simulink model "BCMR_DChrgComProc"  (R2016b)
settings: Solver=FixedStepDiscrete  StartTime=0.0  StopTime=10.0  FixedStep=0.01  RelTol=1e-3  EnableMultiTasking=on
undefined symbols (not defined in the file or in its folder): BCMR_ahBattRatdCpctyBrm_C, BCMR_BattSocErrBsmEna_C, BCMR_eBattRatedEnrgBcp_C, BCMR_G1E0PlatformSwCom_C, BCMR_iMaxChrgCurrPmtdBcp_C, BCMR_numBattTypeBrm_C, BCMR_numComVer2011Brm_C, BCMR_numComVer2015Brm_C, BCMR_tMaxTempPmtdBcp_C, BCMR_uBattRatdPackVoltBcp_C, BCMR_uBattRatdPackVoltBrm_C, BCMR_uMaxChrgCellVoltPmtdBcp_C, BCMR_uMaxPmtDChrgVolt_C
libraries: simulink x32
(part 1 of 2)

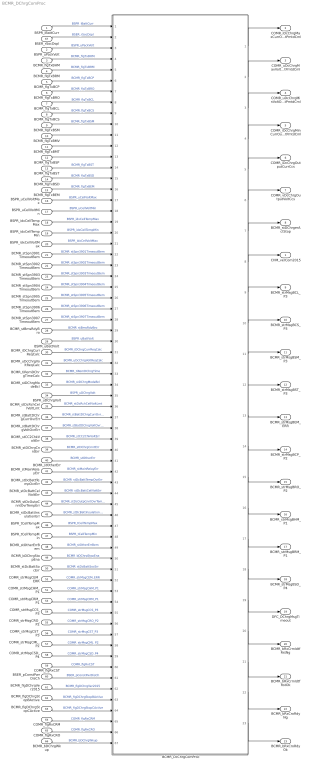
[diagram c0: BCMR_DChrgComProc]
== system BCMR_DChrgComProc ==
  BSPR_iBattCurr : Inport
  BSPR_uPackVolt : Inport  Port=2
  BCMR_flgTxBHM : Inport  Port=3
  BCMR_flgTxBRM : Inport  Port=4
  BCMR_flgTxBCP : Inport  Port=5
  BCMR_flgTxBRO : Inport  Port=6
  BCMR_flgTxBCL : Inport  Port=7
  BCMR_flgTxBCS : Inport  Port=8
  BCMR_flgTxBSM : Inport  Port=9
  BCMR_flgTxBMV : Inport  Port=10
  BCMR_flgTxBMT : Inport  Port=11
  BCMR_flgTxBSP : Inport  Port=12
  BCMR_flgTxBST : Inport  Port=13
  BCMR_flgTxBSD : Inport  Port=14
  BCMR_flgTxBEM : Inport  Port=15
  BSPR_uCellVoltMax : Inport  Port=16
  BSPR_uCellVoltMin : Inport  Port=17
  BSPR_idxCellTempMax : Inport  Port=18
  BSPR_idxCellTempMin : Inport  Port=19
  BSPR_idxCellVoltMax : Inport  Port=20
  BCMR_stSpn3901TimeoutBem : Inport  Port=21
  BCMR_stSpn3902TimeoutBem : Inport  Port=22
  BCMR_stSpn3903TimeoutBem : Inport  Port=23
  BCMR_stSpn3904TimeoutBem : Inport  Port=24
  BCMR_stSpn3905TimeoutBem : Inport  Port=25
  BCMR_stSpn3906TimeoutBem : Inport  Port=26
  BCMR_stSpn3907TimeoutBem : Inport  Port=27
  BCMR_stBmsRdyBro : Inport  Port=28
  BSPR_uBattVolt : Inport  Port=29
  BCMR_iDChrgCurrReqCalc : Inport  Port=30
  BCMR_uDcChrgVoltReqCalc : Inport  Port=31
  BCMR_tiRemDChrgTimeCalc : Inport  Port=32
  BCMR_stDChrgModeBcl : Inport  Port=33
  BSPR_uDChrgVolt : Inport  Port=34
  BCMR_stDcRchCellVoltLmt : Inport  Port=35
  BCMR_stBattDChrgCurrOvrErr : Inport  Port=36
  BCMR_stBattDChrgVoltOvrErr : Inport  Port=37
  BCMR_stCC2ChkVoltErr : Inport  Port=38
  BCMR_stDChrgCnntErr : Inport  Port=39
  BCMR_stOtherErr : Inport  Port=40
  BCMR_stMainRelayErr : Inport  Port=41
  BCMR_stDcBattTempOvrErr : Inport  Port=42
  BCMR_stDcBattCellVoltErr : Inport  Port=43
  BCMR_stDcOutpCnntOvrTempErr : Inport  Port=44
  BCMR_stDcBattInsulationErr : Inport  Port=45
  BSPR_tCellTempMax : Inport  Port=46
  BSPR_tCellTempMin : Inport  Port=47
  BCMR_stOtherErrBem : Inport  Port=48
  BCMR_bDChrgStopEna : Inport  Port=49
  BCMR_stDcBattSocErr : Inport  Port=50
  COMR_strMsgCHM_P1 : Inport  Port=51  OutDataTypeStr=Bus: MSG_CHM_P1
  COMR_strMsgCEM_ERR : Inport  Port=52  OutDataTypeStr=Bus: MSG_CEM_ERR
  COMR_strMsgCRM_P1 : Inport  Port=53  OutDataTypeStr=Bus: MSG_CRM_P1
  COMR_strMsgCCS_P3 : Inport  Port=54  OutDataTypeStr=Bus: MSG_CCS_P3
  COMR_strMsgCRO_P2 : Inport  Port=55  OutDataTypeStr=Bus: MSG_CRO_P2
  COMR_strMsgCST_P3 : Inport  Port=56  OutDataTypeStr=Bus: MSG_CST_P3
  COMR_strMsgCML_P2 : Inport  Port=57  OutDataTypeStr=Bus: MSG_CML_P2
  COMR_strMsgCSD_P4 : Inport  Port=58  OutDataTypeStr=Bus: MSG_CSD_P4
  COMR_flgRxCST : Inport  Port=59
  BSER_pConstPwrDisCh : Inport  Port=60
  BCMR_flgDChrgVer2015 : Inport  Port=61
  BCMR_flgDChrgStopBActive : Inport  Port=62
  BCMR_flgDChrgStopCActive : Inport  Port=63
  COMR_flgRxCRM : Inport  Port=64
  COMR_flgRxCRO : Inport  Port=65
  BCMR_bDChrgWkup : Inport  Port=66
  BSER_rSocDspl : Inport  Port=67
  BCMR_DcChrgComProc : Subsystem
  CHM_verCom2015 : Outport
  COMR_iDcChrgMaxCurrOutputPmtdCml : Outport  Port=2
  COMR_uDcChrgMaxVoltOutputPmtdCml : Outport  Port=3
  COMR_uDcChrgMinVoltOutputPmtdCml : Outport  Port=4
  COMR_iDcChrgMinCurrOutputPmtdCml : Outport  Port=5
  COMR_iDcChrgOutputCurrCcs : Outport  Port=6
  COMR_vDcChrgOutputVoltCcs : Outport  Port=7
  BCMR_stDChrgerActStop : Outport  Port=8
  BCMR_strMsgBCL_P3 : Outport  Port=9  OutDataTypeStr=Bus: MSG_BCL_P3
  BCMR_strMsgBCS_P3 : Outport  Port=10  OutDataTypeStr=Bus: MSG_BCS_P3
  BCMR_strMsgBSM_P3 : Outport  Port=11  OutDataTypeStr=Bus: MSG_BSM_P3
  BCMR_strMsgBST_P3 : Outport  Port=12  OutDataTypeStr=Bus: MSG_BST_P3
  BCMR_strMsgBEM_ERR : Outport  Port=13  OutDataTypeStr=Bus: MSG_BEM_ERR
  BCMR_strMsgBCP_P2 : Outport  Port=14  OutDataTypeStr=Bus: MSG_BCP_P2
  BCMR_strMsgBRO_P2 : Outport  Port=15  OutDataTypeStr=Bus: MSG_BRO_P2
  BCMR_strMsgBHM_P1 : Outport  Port=16  OutDataTypeStr=Bus: MSG_BHM_P1
  BCMR_strMsgBRM_P1 : Outport  Port=17  OutDataTypeStr=Bus: MSG_BRM_P1
  BCMR_strMsgBSD_P4 : Outport  Port=18  OutDataTypeStr=Bus: MSG_BSD_P4
  DFC_DChrgMsgTimeout : Outport  Port=19
  BCMR_bRxCrmIdtfRstNg : Outport  Port=20
  BCMR_bRxCrmIdtfRstOk : Outport  Port=21
  BCMR_bRxCroRdyNg : Outport  Port=22
  BCMR_bRxCroRdyOk : Outport  Port=23
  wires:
  BSPR_iBattCurr/1 -> BCMR_DcChrgComProc/1(BSPR_iBattCurr)  "BSPR_iBattCurr"
  BSPR_uPackVolt/1 -> BCMR_DcChrgComProc/3(BSPR_uPackVolt)  "BSPR_uPackVolt"
  BCMR_flgTxBHM/1 -> BCMR_DcChrgComProc/4(BCMR_flgTxBHM)  "BCMR_flgTxBHM"
  BCMR_flgTxBRM/1 -> BCMR_DcChrgComProc/5(BCMR_flgTxBRM)  "BCMR_flgTxBRM"
  BCMR_flgTxBCP/1 -> BCMR_DcChrgComProc/6(BCMR_flgTxBCP)  "BCMR_flgTxBCP"
  BCMR_flgTxBRO/1 -> BCMR_DcChrgComProc/7(BCMR_flgTxBRO)  "BCMR_flgTxBRO"
  BCMR_flgTxBCL/1 -> BCMR_DcChrgComProc/8(BCMR_flgTxBCL)  "BCMR_flgTxBCL"
  BCMR_flgTxBCS/1 -> BCMR_DcChrgComProc/9(BCMR_flgTxBCS)  "BCMR_flgTxBCS"
  BCMR_flgTxBSM/1 -> BCMR_DcChrgComProc/10(BCMR_flgTxBSM)  "BCMR_flgTxBSM"
  BCMR_flgTxBMV/1 -> BCMR_DcChrgComProc/11(BCMR_flgTxBMV)
  BCMR_flgTxBMT/1 -> BCMR_DcChrgComProc/12(BCMR_flgTxBMT)
  BCMR_flgTxBSP/1 -> BCMR_DcChrgComProc/13(BCMR_flgTxBSP)
  BCMR_flgTxBST/1 -> BCMR_DcChrgComProc/14(BCMR_flgTxBST)  "BCMR_flgTxBST"
  BCMR_flgTxBSD/1 -> BCMR_DcChrgComProc/15(BCMR_flgTxBSD)  "BCMR_flgTxBSD"
  BCMR_flgTxBEM/1 -> BCMR_DcChrgComProc/16(BCMR_flgTxBEM)  "BCMR_flgTxBEM"
  BSPR_uCellVoltMax/1 -> BCMR_DcChrgComProc/17(BSPR_uCellVoltMax)  "BSPR_uCellVoltMax"
  BSPR_uCellVoltMin/1 -> BCMR_DcChrgComProc/18(BSPR_uCellVoltMin)  "BSPR_uCellVoltMin"
  BSPR_idxCellTempMax/1 -> BCMR_DcChrgComProc/19(BSPR_idxBattTempMax)  "BSPR_idxCellTempMax"
  BSPR_idxCellTempMin/1 -> BCMR_DcChrgComProc/20(BSPR_idxBattTempMin)  "BSPR_idxCellTempMin"
  BSPR_idxCellVoltMax/1 -> BCMR_DcChrgComProc/21(BSPR_idxCellVoltMax)  "BSPR_idxCellVoltMax"
  BCMR_stSpn3901TimeoutBem/1 -> BCMR_DcChrgComProc/22(BCMR_stSpn3901TimeoutBem)  "BCMR_stSpn3901TimeoutBem"
  BCMR_stSpn3902TimeoutBem/1 -> BCMR_DcChrgComProc/23(BCMR_stSpn3902TimeoutBem)  "BCMR_stSpn3902TimeoutBem"
  BCMR_stSpn3903TimeoutBem/1 -> BCMR_DcChrgComProc/24(BCMR_stSpn3903TimeoutBem)  "BCMR_stSpn3903TimeoutBem"
  BCMR_stSpn3904TimeoutBem/1 -> BCMR_DcChrgComProc/25(BCMR_stSpn3904TimeoutBem)  "BCMR_stSpn3904TimeoutBem"
  BCMR_stSpn3905TimeoutBem/1 -> BCMR_DcChrgComProc/26(BCMR_stSpn3905TimeoutBem)  "BCMR_stSpn3905TimeoutBem"
  BCMR_stSpn3906TimeoutBem/1 -> BCMR_DcChrgComProc/27(BCMR_stSpn3906TimeoutBem)  "BCMR_stSpn3906TimeoutBem"
  BCMR_stSpn3907TimeoutBem/1 -> BCMR_DcChrgComProc/28(BCMR_stSpn3907TimeoutBem)  "BCMR_stSpn3907TimeoutBem"
  BCMR_stBmsRdyBro/1 -> BCMR_DcChrgComProc/29(BCMR_stBmsRdyBro)  "BCMR_stBmsRdyBro"
  BSPR_uBattVolt/1 -> BCMR_DcChrgComProc/30(BSPR_uBattVolt)  "BSPR_uBattVolt"
  BCMR_iDChrgCurrReqCalc/1 -> BCMR_DcChrgComProc/31(BCMR_iDChrgCurrReqCalc)  "BCMR_iDChrgCurrReqCalc"
  BCMR_uDcChrgVoltReqCalc/1 -> BCMR_DcChrgComProc/32(BCMR_uDcChrgVoltReqCalc)  "BCMR_uDcChrgVoltReqCalc"
  BCMR_tiRemDChrgTimeCalc/1 -> BCMR_DcChrgComProc/33(BCMR_tiRemDChrgTime)  "BCMR_tiRemDChrgTime"
  BCMR_stDChrgModeBcl/1 -> BCMR_DcChrgComProc/34(BCMR_stDChrgModeBcl)  "BCMR_stDChrgModeBcl"
  BSPR_uDChrgVolt/1 -> BCMR_DcChrgComProc/35(BSPR_uDChrgVolt)  "BSPR_uDChrgVolt"
  BCMR_stDcRchCellVoltLmt/1 -> BCMR_DcChrgComProc/36(BCMR_stDcRchCellVoltLmt)  "BCMR_stDcRchCellVoltLmt"
  BCMR_stBattDChrgCurrOvrErr/1 -> BCMR_DcChrgComProc/37(BCMR_stBattDChrgCurrOvrErr)  "BCMR_stBattDChrgCurrOvrErr"
  BCMR_stBattDChrgVoltOvrErr/1 -> BCMR_DcChrgComProc/38(BCMR_stBattDChrgVoltOvrErr)  "BCMR_stBattDChrgVoltOvrErr"
  BCMR_stCC2ChkVoltErr/1 -> BCMR_DcChrgComProc/39(BCMR_stCC2ChkVoltErr)  "BCMR_stCC2ChkVoltErr"
  BCMR_stDChrgCnntErr/1 -> BCMR_DcChrgComProc/40(BCMR_stDChrgCnntErr)  "BCMR_stDChrgCnntErr"
  BCMR_stOtherErr/1 -> BCMR_DcChrgComProc/41(BCMR_stOtherErr)  "BCMR_stOtherErr"
  BCMR_stMainRelayErr/1 -> BCMR_DcChrgComProc/42(BCMR_stMainRelayErr)  "BCMR_stMainRelayErr"
  BCMR_stDcBattTempOvrErr/1 -> BCMR_DcChrgComProc/43(BCMR_stDcBattTempOvrErr)  "BCMR_stDcBattTempOvrErr"
  BCMR_stDcBattCellVoltErr/1 -> BCMR_DcChrgComProc/44(BCMR_stDcBattCellVoltErr)  "BCMR_stDcBattCellVoltErr"
  BCMR_stDcOutpCnntOvrTempErr/1 -> BCMR_DcChrgComProc/45(BCMR_stDcOutpCnntOvrTempErr)  "BCMR_stDcOutpCnntOvrTempErr"
  BCMR_stDcBattInsulationErr/1 -> BCMR_DcChrgComProc/46(BCMR_stDcBattInsulationErr)  "BCMR_stDcBattInsulationErr"
  BSPR_tCellTempMax/1 -> BCMR_DcChrgComProc/47(BSPR_tBattTempMax)  "BSPR_tCellTempMax"
  BSPR_tCellTempMin/1 -> BCMR_DcChrgComProc/48(BSPR_tBattTempMin)  "BSPR_tCellTempMin"
  BCMR_DcChrgComProc/1(COMR_iDcChrgMaxCurrOutputPmtdCml) -> COMR_iDcChrgMaxCurrOutputPmtdCml/1
  BCMR_DcChrgComProc/2(COMR_uDcChrgMaxVoltOutputPmtdCml) -> COMR_uDcChrgMaxVoltOutputPmtdCml/1
  BCMR_DcChrgComProc/3(COMR_uDcChrgMinVoltOutputPmtdCml) -> COMR_uDcChrgMinVoltOutputPmtdCml/1
  BCMR_DcChrgComProc/4(COMR_iDcChrgMinCurrOutputPmtdCml) -> COMR_iDcChrgMinCurrOutputPmtdCml/1
  BCMR_DcChrgComProc/5(COMR_iDcChrgOutputCurrCcs) -> COMR_iDcChrgOutputCurrCcs/1
  BCMR_DcChrgComProc/6(COMR_vDcChrgOutputVoltCcs) -> COMR_vDcChrgOutputVoltCcs/1
  BCMR_DcChrgComProc/7(BCMR_stDChrgerActStop) -> BCMR_stDChrgerActStop/1
  BCMR_stOtherErrBem/1 -> BCMR_DcChrgComProc/49(BCMR_stOtherErrBem)  "BCMR_stOtherErrBem"
  BCMR_DcChrgComProc/8(BCMR_verDChrgCom2015) -> CHM_verCom2015/1
  BCMR_bDChrgStopEna/1 -> BCMR_DcChrgComProc/50(BCMR_bDChrgStopEna)  "BCMR_bDChrgStopEna"
  BCMR_stDcBattSocErr/1 -> BCMR_DcChrgComProc/51(BCMR_stDcBattSocErr)  "BCMR_stDcBattSocErr"
  COMR_strMsgCSD_P4/1 -> BCMR_DcChrgComProc/59(COMR_strRxCSD)  "COMR_strMsgCSD_P4"
  COMR_strMsgCML_P2/1 -> BCMR_DcChrgComProc/58(COMR_strRxCML)  "COMR_strMsgCML_P2"
  COMR_strMsgCST_P3/1 -> BCMR_DcChrgComProc/57(COMR_strRxCST)  "COMR_strMsgCST_P3"
  COMR_strMsgCRO_P2/1 -> BCMR_DcChrgComProc/56(COMR_strRxCRO)  "COMR_strMsgCRO_P2"
  COMR_strMsgCCS_P3/1 -> BCMR_DcChrgComProc/55(COMR_strRxCCS)  "COMR_strMsgCCS_P3"
  COMR_strMsgCRM_P1/1 -> BCMR_DcChrgComProc/54(COMR_strRxCRM)  "COMR_strMsgCRM_P1"
  COMR_strMsgCEM_ERR/1 -> BCMR_DcChrgComProc/52(COMR_strRxCEM)  "COMR_strMsgCEM_ERR"
  COMR_strMsgCHM_P1/1 -> BCMR_DcChrgComProc/53(COMR_strRxCHM)  "COMR_strMsgCHM_P1"
  BCMR_DcChrgComProc/9(BCMR_strMsgBCL_P3) -> BCMR_strMsgBCL_P3/1
  BCMR_DcChrgComProc/10(BCMR_strMsgBCS_P3) -> BCMR_strMsgBCS_P3/1
  BCMR_DcChrgComProc/11(BCMR_strMsgBSM_P3) -> BCMR_strMsgBSM_P3/1
  BCMR_DcChrgComProc/12(BCMR_strMsgBST_P3) -> BCMR_strMsgBST_P3/1
  BCMR_DcChrgComProc/13(BCMR_strMsgBEM_ERR) -> BCMR_strMsgBEM_ERR/1
  BCMR_DcChrgComProc/14(BCMR_strMsgBCP_P2) -> BCMR_strMsgBCP_P2/1
  BCMR_DcChrgComProc/15(BCMR_strMsgBRO_P2) -> BCMR_strMsgBRO_P2/1
  BCMR_DcChrgComProc/16(BCMR_strMsgBHM_P1) -> BCMR_strMsgBHM_P1/1
  BCMR_DcChrgComProc/17(BCMR_strMsgBRM_P1) -> BCMR_strMsgBRM_P1/1
  BCMR_DcChrgComProc/18(BCMR_strMsgBSD_P4) -> BCMR_strMsgBSD_P4/1
  BCMR_DcChrgComProc/19(DFC_DChrgMsgTimeout) -> DFC_DChrgMsgTimeout/1
  COMR_flgRxCST/1 -> BCMR_DcChrgComProc/60(COMR_flgRxCST)  "COMR_flgRxCST"
  BSER_pConstPwrDisCh/1 -> BCMR_DcChrgComProc/61(BSER_pConstPwrDisCh)  "BSER_pConstPwrDisCh"
  BCMR_flgDChrgVer2015/1 -> BCMR_DcChrgComProc/62(BCMR_flgDChrgVer2015)  "BCMR_flgDChrgVer2015"
  BCMR_flgDChrgStopBActive/1 -> BCMR_DcChrgComProc/63(BCMR_flgDChrgStopBActive)  "BCMR_flgDChrgStopBActive"
  BCMR_flgDChrgStopCActive/1 -> BCMR_DcChrgComProc/64(BCMR_flgDChrgStopCActive)  "BCMR_flgDChrgStopCActive"
  COMR_flgRxCRM/1 -> BCMR_DcChrgComProc/65(COMR_flgRxCRM)  "COMR_flgRxCRM"
  COMR_flgRxCRO/1 -> BCMR_DcChrgComProc/66(COMR_flgRxCRO)  "COMR_flgRxCRO"
  BCMR_DcChrgComProc/20(BCMR_bRxCrmIdtfRstNg) -> BCMR_bRxCrmIdtfRstNg/1
  BCMR_DcChrgComProc/21(BCMR_bRxCrmIdtfRstOk) -> BCMR_bRxCrmIdtfRstOk/1
  BCMR_DcChrgComProc/23(BCMR_bRxCroRdyOk) -> BCMR_bRxCroRdyOk/1
  BCMR_DcChrgComProc/22(BCMR_bRxCroRdyNg) -> BCMR_bRxCroRdyNg/1
  BCMR_bDChrgWkup/1 -> BCMR_DcChrgComProc/67(BCMR_bDChrgWkup)  "BCMR_bDChrgWkup"
  BSER_rSocDspl/1 -> BCMR_DcChrgComProc/2(BSER_rSocDspl)  "BSER_rSocDspl"

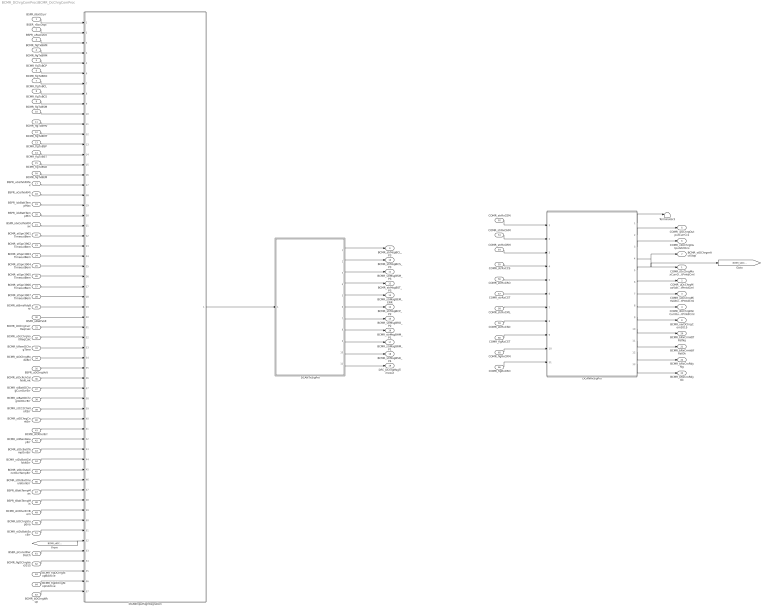
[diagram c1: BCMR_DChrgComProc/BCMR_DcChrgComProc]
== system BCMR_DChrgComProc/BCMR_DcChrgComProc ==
  BSPR_iBattCurr : Inport
  BSER_rSocDspl : Inport  Port=2
  BSPR_uPackVolt : Inport  Port=3
  BCMR_flgTxBHM : Inport  Port=4
  BCMR_flgTxBRM : Inport  Port=5
  BCMR_flgTxBCP : Inport  Port=6
  BCMR_flgTxBRO : Inport  Port=7
  BCMR_flgTxBCL : Inport  Port=8
  BCMR_flgTxBCS : Inport  Port=9
  BCMR_flgTxBSM : Inport  Port=10
  BCMR_flgTxBMV : Inport  Port=11
  BCMR_flgTxBMT : Inport  Port=12
  BCMR_flgTxBSP : Inport  Port=13
  BCMR_flgTxBST : Inport  Port=14
  BCMR_flgTxBSD : Inport  Port=15
  BCMR_flgTxBEM : Inport  Port=16
  BSPR_uCellVoltMax : Inport  Port=17
  BSPR_uCellVoltMin : Inport  Port=18
  BSPR_idxBattTempMax : Inport  Port=19
  BSPR_idxBattTempMin : Inport  Port=20
  BSPR_idxCellVoltMax : Inport  Port=21
  BCMR_stSpn3901TimeoutBem : Inport  Port=22
  BCMR_stSpn3902TimeoutBem : Inport  Port=23
  BCMR_stSpn3903TimeoutBem : Inport  Port=24
  BCMR_stSpn3904TimeoutBem : Inport  Port=25
  BCMR_stSpn3905TimeoutBem : Inport  Port=26
  BCMR_stSpn3906TimeoutBem : Inport  Port=27
  BCMR_stSpn3907TimeoutBem : Inport  Port=28
  BCMR_stBmsRdyBro : Inport  Port=29
  BSPR_uBattVolt : Inport  Port=30
  BCMR_iDChrgCurrReqCalc : Inport  Port=31
  BCMR_uDcChrgVoltReqCalc : Inport  Port=32
  BCMR_tiRemDChrgTime : Inport  Port=33
  BCMR_stDChrgModeBcl : Inport  Port=34
  BSPR_uDChrgVolt : Inport  Port=35
  BCMR_stDcRchCellVoltLmt : Inport  Port=36
  BCMR_stBattDChrgCurrOvrErr : Inport  Port=37
  BCMR_stBattDChrgVoltOvrErr : Inport  Port=38
  BCMR_stCC2ChkVoltErr : Inport  Port=39
  BCMR_stDChrgCnntErr : Inport  Port=40
  BCMR_stOtherErr : Inport  Port=41
  BCMR_stMainRelayErr : Inport  Port=42
  BCMR_stDcBattTempOvrErr : Inport  Port=43
  BCMR_stDcBattCellVoltErr : Inport  Port=44
  BCMR_stDcOutpCnntOvrTempErr : Inport  Port=45
  BCMR_stDcBattInsulationErr : Inport  Port=46
  BSPR_tBattTempMax : Inport  Port=47
  BSPR_tBattTempMin : Inport  Port=48
  BCMR_stOtherErrBem : Inport  Port=49
  BCMR_bDChrgStopEna : Inport  Port=50
  BCMR_stDcBattSocErr : Inport  Port=51
  COMR_strRxCEM : Inport  Port=52  OutDataTypeStr=Bus: MSG_CEM_ERR
  COMR_strRxCHM : Inport  Port=53  OutDataTypeStr=Bus: MSG_CHM_P1
  COMR_strRxCRM : Inport  Port=54  OutDataTypeStr=Bus: MSG_CRM_P1
  COMR_strRxCCS : Inport  Port=55  OutDataTypeStr=Bus: MSG_CCS_P3
  COMR_strRxCRO : Inport  Port=56  OutDataTypeStr=Bus: MSG_CRO_P2
  COMR_strRxCST : Inport  Port=57  OutDataTypeStr=Bus: MSG_CST_P3
  COMR_strRxCML : Inport  Port=58  OutDataTypeStr=Bus: MSG_CML_P2
  COMR_strRxCSD : Inport  Port=59  OutDataTypeStr=Bus: MSG_CSD_P4
  COMR_flgRxCST : Inport  Port=60
  BSER_pConstPwrDisCh : Inport  Port=61
  BCMR_flgDChrgVer2015 : Inport  Port=62
  BCMR_flgDChrgStopBActive : Inport  Port=63
  BCMR_flgDChrgStopCActive : Inport  Port=64
  COMR_flgRxCRM : Inport  Port=65
  COMR_flgRxCRO : Inport  Port=66
  BCMR_bDChrgWkup : Inport  Port=67
  DCANInputSigIntegration : Subsystem
  DCANRxSigPro : Subsystem
  DCANTxSigPro : Subsystem
  Terminator3 : Terminator
  COMR_iDcChrgMaxCurrOutputPmtdCml : Outport
  COMR_uDcChrgMaxVoltOutputPmtdCml : Outport  Port=2
  COMR_uDcChrgMinVoltOutputPmtdCml : Outport  Port=3
  COMR_iDcChrgMinCurrOutputPmtdCml : Outport  Port=4
  COMR_iDcChrgOutputCurrCcs : Outport  Port=5
  COMR_vDcChrgOutputVoltCcs : Outport  Port=6
  BCMR_stDChrgerActStop : Outport  Port=7
  BCMR_verDChrgCom2015 : Outport  Port=8
  BCMR_strMsgBCL_P3 : Outport  Port=9  OutDataTypeStr=Bus: MSG_BCL_P3
  BCMR_strMsgBCS_P3 : Outport  Port=10  OutDataTypeStr=Bus: MSG_BCS_P3
  BCMR_strMsgBSM_P3 : Outport  Port=11  OutDataTypeStr=Bus: MSG_BSM_P3
  BCMR_strMsgBST_P3 : Outport  Port=12  OutDataTypeStr=Bus: MSG_BST_P3
  BCMR_strMsgBEM_ERR : Outport  Port=13  OutDataTypeStr=Bus: MSG_BEM_ERR
  BCMR_strMsgBCP_P2 : Outport  Port=14  OutDataTypeStr=Bus: MSG_BCP_P2
  BCMR_strMsgBRO_P2 : Outport  Port=15  OutDataTypeStr=Bus: MSG_BRO_P2
  BCMR_strMsgBHM_P1 : Outport  Port=16  OutDataTypeStr=Bus: MSG_BHM_P1
  BCMR_strMsgBRM_P1 : Outport  Port=17  OutDataTypeStr=Bus: MSG_BRM_P1
  BCMR_strMsgBSD_P4 : Outport  Port=18  OutDataTypeStr=Bus: MSG_BSD_P4
  DFC_DChrgMsgTimeout : Outport  Port=19
  BCMR_bRxCrmIdtfRstNg : Outport  Port=20
  BCMR_bRxCrmIdtfRstOk : Outport  Port=21
  BCMR_bRxCroRdyNg : Outport  Port=22
  BCMR_bRxCroRdyOk : Outport  Port=23
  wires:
  COMR_strRxCEM/1 -> DCANRxSigPro/1(COMR_strRxCEM)
  COMR_strRxCHM/1 -> DCANRxSigPro/2(COMR_strRxCHM)
  COMR_strRxCRM/1 -> DCANRxSigPro/3(COMR_strRxCRM)
  COMR_strRxCCS/1 -> DCANRxSigPro/4(COMR_strRxCCS)
  COMR_strRxCRO/1 -> DCANRxSigPro/5(COMR_strRxCRO)
  COMR_strRxCST/1 -> DCANRxSigPro/6(COMR_strRxCST)
  COMR_strRxCML/1 -> DCANRxSigPro/7(COMR_strRxCML)
  COMR_strRxCSD/1 -> DCANRxSigPro/8(COMR_strRxCSD)
  DCANRxSigPro/2(COMR_iDcChrgOutputCurrCcs) -> COMR_iDcChrgOutputCurrCcs/1
  DCANRxSigPro/3(COMR_vDcChrgOutputVoltCcs) -> COMR_vDcChrgOutputVoltCcs/1
  DCANRxSigPro/4(BCMR_stDChrgerActStop) -> [BCMR_stDChrgerActStop], BCMR_stDChrgerActStop/1
  DCANRxSigPro/5(COMR_iDcChrgMaxCurrOutputPmtdCml) -> COMR_iDcChrgMaxCurrOutputPmtdCml/1
  DCANRxSigPro/6(COMR_uDcChrgMaxVoltOutputPmtdCml) -> COMR_uDcChrgMaxVoltOutputPmtdCml/1
  DCANRxSigPro/7(COMR_uDcChrgMinVoltOutputPmtdCml) -> COMR_uDcChrgMinVoltOutputPmtdCml/1
  DCANRxSigPro/8(COMR_iDcChrgMinCurrOutputPmtdCml) -> COMR_iDcChrgMinCurrOutputPmtdCml/1
  DCANRxSigPro/9(BCMR_verDChrgCom2015) -> BCMR_verDChrgCom2015/1
  BSPR_iBattCurr/1 -> DCANInputSigIntegration/1(BSPR_iBattCurr)
  BSER_rSocDspl/1 -> DCANInputSigIntegration/2(BSER_rSocDspl)
  BSPR_uPackVolt/1 -> DCANInputSigIntegration/3(BSPR_uPackVolt)
  BCMR_flgTxBHM/1 -> DCANInputSigIntegration/4(BCMR_flgTxBHM)
  BCMR_flgTxBRM/1 -> DCANInputSigIntegration/5(BCMR_flgTxBRM)
  BCMR_flgTxBCP/1 -> DCANInputSigIntegration/6(BCMR_flgTxBCP)
  BCMR_flgTxBRO/1 -> DCANInputSigIntegration/7(BCMR_flgTxBRO)
  BCMR_flgTxBCL/1 -> DCANInputSigIntegration/8(BCMR_flgTxBCL)
  BCMR_flgTxBCS/1 -> DCANInputSigIntegration/9(BCMR_flgTxBCS)
  BCMR_flgTxBSM/1 -> DCANInputSigIntegration/10(BCMR_flgTxBSM)
  BCMR_flgTxBMV/1 -> DCANInputSigIntegration/11(BCMR_flgTxBMV)
  BCMR_flgTxBMT/1 -> DCANInputSigIntegration/12(BCMR_flgTxBMT)
  BCMR_flgTxBSP/1 -> DCANInputSigIntegration/13(BCMR_flgTxBSP)
  BCMR_flgTxBST/1 -> DCANInputSigIntegration/14(BCMR_flgTxBST)
  BCMR_flgTxBSD/1 -> DCANInputSigIntegration/15(BCMR_flgTxBSD)
  BCMR_flgTxBEM/1 -> DCANInputSigIntegration/16(BCMR_flgTxBEM)
  BSPR_uCellVoltMax/1 -> DCANInputSigIntegration/17(BSPR_uCellVoltMax)
  BSPR_uCellVoltMin/1 -> DCANInputSigIntegration/18(BSPR_uCellVoltMin)
  BSPR_idxBattTempMax/1 -> DCANInputSigIntegration/19(BSPR_idxBattTempMax)
  BSPR_idxBattTempMin/1 -> DCANInputSigIntegration/20(BSPR_idxBattTempMin)
  BSPR_idxCellVoltMax/1 -> DCANInputSigIntegration/21(BSPR_idxCellVoltMax)
  BCMR_stSpn3901TimeoutBem/1 -> DCANInputSigIntegration/22(BCMR_stSpn3901TimeoutBem)
  BCMR_stSpn3902TimeoutBem/1 -> DCANInputSigIntegration/23(BCMR_stSpn3902TimeoutBem)
  BCMR_stSpn3903TimeoutBem/1 -> DCANInputSigIntegration/24(BCMR_stSpn3903TimeoutBem)
  BCMR_stSpn3904TimeoutBem/1 -> DCANInputSigIntegration/25(BCMR_stSpn3904TimeoutBem)
  BCMR_stSpn3905TimeoutBem/1 -> DCANInputSigIntegration/26(BCMR_stSpn3905TimeoutBem)
  BCMR_stSpn3906TimeoutBem/1 -> DCANInputSigIntegration/27(BCMR_stSpn3906TimeoutBem)
  BCMR_stSpn3907TimeoutBem/1 -> DCANInputSigIntegration/28(BCMR_stSpn3907TimeoutBem)
  BCMR_stBmsRdyBro/1 -> DCANInputSigIntegration/29(BCMR_stBmsRdyBro)
  BSPR_uBattVolt/1 -> DCANInputSigIntegration/30(BSPR_uBattVolt)
  BCMR_iDChrgCurrReqCalc/1 -> DCANInputSigIntegration/31(BCMR_iDChrgCurrReqCalc)
  BCMR_uDcChrgVoltReqCalc/1 -> DCANInputSigIntegration/32(BCMR_uDcChrgVoltReqCalc)
  BCMR_tiRemDChrgTime/1 -> DCANInputSigIntegration/33(BCMR_tiRemDChrgTime)
  BCMR_stDChrgModeBcl/1 -> DCANInputSigIntegration/34(BCMR_stDChrgModeBcl)
  BSPR_uDChrgVolt/1 -> DCANInputSigIntegration/35(BSPR_uDChrgVolt)
  BCMR_stDcRchCellVoltLmt/1 -> DCANInputSigIntegration/36(BCMR_stDcRchCellVoltLmt)
  BCMR_stBattDChrgCurrOvrErr/1 -> DCANInputSigIntegration/37(BCMR_stBattDChrgCurrOvrErr)
  BCMR_stBattDChrgVoltOvrErr/1 -> DCANInputSigIntegration/38(BCMR_stBattDChrgVoltOvrErr)
  BCMR_stCC2ChkVoltErr/1 -> DCANInputSigIntegration/39(BCMR_stCC2ChkVoltErr)
  BCMR_stDChrgCnntErr/1 -> DCANInputSigIntegration/40(BCMR_stDChrgCnntErr)
  BCMR_stOtherErr/1 -> DCANInputSigIntegration/41(BCMR_stOtherErr)
  BCMR_stMainRelayErr/1 -> DCANInputSigIntegration/42(BCMR_stMainRelayErr)
  BCMR_stDcBattTempOvrErr/1 -> DCANInputSigIntegration/43(BCMR_stDcBattTempOvrErr)
  BCMR_stDcBattCellVoltErr/1 -> DCANInputSigIntegration/44(BCMR_stDcBattCellVoltErr)
  BCMR_stDcOutpCnntOvrTempErr/1 -> DCANInputSigIntegration/45(BCMR_stDcOutpCnntOvrTempErr)
  BCMR_stDcBattInsulationErr/1 -> DCANInputSigIntegration/46(BCMR_stDcBattInsulationErr)
  BSPR_tBattTempMax/1 -> DCANInputSigIntegration/47(BSPR_tBattTempMax)
  BSPR_tBattTempMin/1 -> DCANInputSigIntegration/48(BSPR_tBattTempMin)
  DCANInputSigIntegration/1(DCAN_DataFlow) -> DCANTxSigPro/1(DCAN_DataFlow)
  BCMR_stOtherErrBem/1 -> DCANInputSigIntegration/49(BCMR_stOtherErrBem)
  BCMR_bDChrgStopEna/1 -> DCANInputSigIntegration/50(BCMR_bDChrgStopEna)
  BCMR_stDcBattSocErr/1 -> DCANInputSigIntegration/51(BCMR_stDcBattSocErr)
  [BCMR_stDChrgerActStop] -> DCANInputSigIntegration/52(BCMR_stDChrgerActStop)
  DCANTxSigPro/1(BCMR_strMsgBCL_P3) -> BCMR_strMsgBCL_P3/1
  DCANTxSigPro/2(BCMR_strMsgBCS_P3) -> BCMR_strMsgBCS_P3/1
  DCANTxSigPro/3(BCMR_strMsgBSM_P3) -> BCMR_strMsgBSM_P3/1
  DCANTxSigPro/4(BCMR_strMsgBST_P3) -> BCMR_strMsgBST_P3/1
  DCANTxSigPro/5(BCMR_strMsgBEM_ERR) -> BCMR_strMsgBEM_ERR/1
  DCANTxSigPro/7(BCMR_strMsgBRO_P2) -> BCMR_strMsgBRO_P2/1
  DCANTxSigPro/8(BCMR_strMsgBHM_P1) -> BCMR_strMsgBHM_P1/1
  DCANTxSigPro/9(BCMR_strMsgBRM_P1) -> BCMR_strMsgBRM_P1/1
  DCANTxSigPro/10(BCMR_strMsgBSD_P4) -> BCMR_strMsgBSD_P4/1
  DCANTxSigPro/11(DFC_DChrgMsgTimeout) -> DFC_DChrgMsgTimeout/1
  COMR_flgRxCST/1 -> DCANRxSigPro/9(COMR_flgRxCST)
  BSER_pConstPwrDisCh/1 -> DCANInputSigIntegration/53(BSER_pConstPwrDisCh)
  BCMR_flgDChrgVer2015/1 -> DCANInputSigIntegration/54(BCMR_verDChrgCom2015)
  DCANTxSigPro/6(BCMR_strMsgBCP_P2) -> BCMR_strMsgBCP_P2/1
  BCMR_flgDChrgStopBActive/1 -> DCANInputSigIntegration/55(BCMR_flgDChrgStopBActive)
  BCMR_flgDChrgStopCActive/1 -> DCANInputSigIntegration/56(BCMR_flgDChrgStopCActive)
  COMR_flgRxCRM/1 -> DCANRxSigPro/10(COMR_flgRxCRM)
  COMR_flgRxCRO/1 -> DCANRxSigPro/11(COMR_flgRxCRO)
  DCANRxSigPro/10(BCMR_bRxCrmIdtfRstNg) -> BCMR_bRxCrmIdtfRstNg/1
  DCANRxSigPro/11(BCMR_bRxCrmIdtfRstOk) -> BCMR_bRxCrmIdtfRstOk/1
  DCANRxSigPro/12(BCMR_bRxCroRdyNg) -> BCMR_bRxCroRdyNg/1
  DCANRxSigPro/13(BCMR_bRxCroRdyOk) -> BCMR_bRxCroRdyOk/1
  BCMR_bDChrgWkup/1 -> DCANInputSigIntegration/57(BCMR_bDChrgWkup)
  DCANRxSigPro/1(DCAN_RxDataFlow) -> Terminator3/1

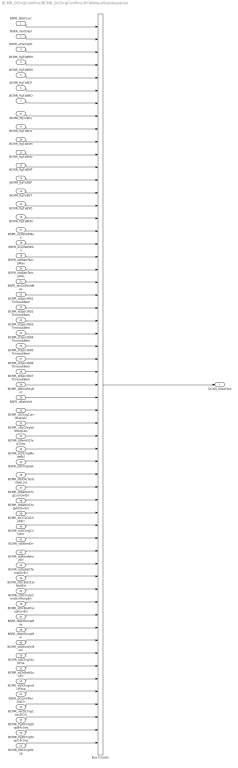
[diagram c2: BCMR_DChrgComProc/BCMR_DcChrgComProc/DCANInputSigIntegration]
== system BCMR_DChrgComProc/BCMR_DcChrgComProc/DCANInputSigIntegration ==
  BSPR_iBattCurr : Inport
  BSER_rSocDspl : Inport  Port=2
  BSPR_uPackVolt : Inport  Port=3
  BCMR_flgTxBHM : Inport  Port=4
  BCMR_flgTxBRM : Inport  Port=5
  BCMR_flgTxBCP : Inport  Port=6
  BCMR_flgTxBRO : Inport  Port=7
  BCMR_flgTxBCL : Inport  Port=8
  BCMR_flgTxBCS : Inport  Port=9
  BCMR_flgTxBSM : Inport  Port=10
  BCMR_flgTxBMV : Inport  Port=11
  BCMR_flgTxBMT : Inport  Port=12
  BCMR_flgTxBSP : Inport  Port=13
  BCMR_flgTxBST : Inport  Port=14
  BCMR_flgTxBSD : Inport  Port=15
  BCMR_flgTxBEM : Inport  Port=16
  BSPR_uCellVoltMax : Inport  Port=17
  BSPR_uCellVoltMin : Inport  Port=18
  BSPR_idxBattTempMax : Inport  Port=19
  BSPR_idxBattTempMin : Inport  Port=20
  BSPR_idxCellVoltMax : Inport  Port=21
  BCMR_stSpn3901TimeoutBem : Inport  Port=22
  BCMR_stSpn3902TimeoutBem : Inport  Port=23
  BCMR_stSpn3903TimeoutBem : Inport  Port=24
  BCMR_stSpn3904TimeoutBem : Inport  Port=25
  BCMR_stSpn3905TimeoutBem : Inport  Port=26
  BCMR_stSpn3906TimeoutBem : Inport  Port=27
  BCMR_stSpn3907TimeoutBem : Inport  Port=28
  BCMR_stBmsRdyBro : Inport  Port=29
  BSPR_uBattVolt : Inport  Port=30
  BCMR_iDChrgCurrReqCalc : Inport  Port=31
  BCMR_uDcChrgVoltReqCalc : Inport  Port=32
  BCMR_tiRemDChrgTime : Inport  Port=33
  BCMR_stDChrgModeBcl : Inport  Port=34
  BSPR_uDChrgVolt : Inport  Port=35
  BCMR_stDcRchCellVoltLmt : Inport  Port=36
  BCMR_stBattDChrgCurrOvrErr : Inport  Port=37
  BCMR_stBattDChrgVoltOvrErr : Inport  Port=38
  BCMR_stCC2ChkVoltErr : Inport  Port=39
  BCMR_stDChrgCnntErr : Inport  Port=40
  BCMR_stOtherErr : Inport  Port=41
  BCMR_stMainRelayErr : Inport  Port=42
  BCMR_stDcBattTempOvrErr : Inport  Port=43
  BCMR_stDcBattCellVoltErr : Inport  Port=44
  BCMR_stDcOutpCnntOvrTempErr : Inport  Port=45
  BCMR_stDcBattInsulationErr : Inport  Port=46
  BSPR_tBattTempMax : Inport  Port=47
  BSPR_tBattTempMin : Inport  Port=48
  BCMR_stOtherErrBem : Inport  Port=49
  BCMR_bDChrgStopEna : Inport  Port=50
  BCMR_stDcBattSocErr : Inport  Port=51
  BCMR_stDChrgerActStop : Inport  Port=52
  BSER_pConstPwrDisCh : Inport  Port=53
  BCMR_verDChrgCom2015 : Inport  Port=54
  BCMR_flgDChrgStopBActive : Inport  Port=55
  BCMR_flgDChrgStopCActive : Inport  Port=56
  BCMR_bDChrgWkup : Inport  Port=57
  Bus Creator : BusCreator  Inputs=57
  DCAN_DataFlow : Outport
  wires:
  Bus Creator/1 -> DCAN_DataFlow/1
  BCMR_stSpn3903TimeoutBem/1 -> Bus Creator/24
  BCMR_stMainRelayErr/1 -> Bus Creator/42
  BSER_rSocDspl/1 -> Bus Creator/2
  BCMR_flgTxBMV/1 -> Bus Creator/11
  BSPR_uCellVoltMin/1 -> Bus Creator/18
  BCMR_flgTxBSP/1 -> Bus Creator/13
  BCMR_stSpn3905TimeoutBem/1 -> Bus Creator/26
  BCMR_stSpn3902TimeoutBem/1 -> Bus Creator/23
  BSPR_uDChrgVolt/1 -> Bus Creator/35
  BCMR_stDcBattTempOvrErr/1 -> Bus Creator/43
  BCMR_flgTxBSM/1 -> Bus Creator/10
  BSPR_iBattCurr/1 -> Bus Creator/1
  BCMR_flgTxBCP/1 -> Bus Creator/6
  BCMR_stBmsRdyBro/1 -> Bus Creator/29
  BCMR_tiRemDChrgTime/1 -> Bus Creator/33
  BCMR_stDcBattInsulationErr/1 -> Bus Creator/46
  BCMR_iDChrgCurrReqCalc/1 -> Bus Creator/31
  BSPR_uCellVoltMax/1 -> Bus Creator/17
  BSPR_idxBattTempMax/1 -> Bus Creator/19
  BCMR_stDcBattCellVoltErr/1 -> Bus Creator/44
  BSPR_uPackVolt/1 -> Bus Creator/3
  BCMR_stOtherErr/1 -> Bus Creator/41
  BCMR_flgTxBCS/1 -> Bus Creator/9
  BCMR_flgTxBRM/1 -> Bus Creator/5
  BCMR_flgTxBEM/1 -> Bus Creator/16
  BSPR_idxBattTempMin/1 -> Bus Creator/20
  BCMR_stBattDChrgCurrOvrErr/1 -> Bus Creator/37
  BCMR_flgTxBCL/1 -> Bus Creator/8
  BCMR_stCC2ChkVoltErr/1 -> Bus Creator/39
  BCMR_stDChrgCnntErr/1 -> Bus Creator/40
  BCMR_flgTxBSD/1 -> Bus Creator/15
  BCMR_stSpn3901TimeoutBem/1 -> Bus Creator/22
  BCMR_flgTxBHM/1 -> Bus Creator/4
  BCMR_stDChrgModeBcl/1 -> Bus Creator/34
  BCMR_stSpn3904TimeoutBem/1 -> Bus Creator/25
  BCMR_stDcRchCellVoltLmt/1 -> Bus Creator/36
  BCMR_flgTxBRO/1 -> Bus Creator/7
  BCMR_stSpn3906TimeoutBem/1 -> Bus Creator/27
  BCMR_stDcOutpCnntOvrTempErr/1 -> Bus Creator/45
  BSPR_tBattTempMax/1 -> Bus Creator/47
  BCMR_flgTxBST/1 -> Bus Creator/14
  BSPR_tBattTempMin/1 -> Bus Creator/48
  BCMR_stSpn3907TimeoutBem/1 -> Bus Creator/28
  BCMR_stBattDChrgVoltOvrErr/1 -> Bus Creator/38
  BCMR_uDcChrgVoltReqCalc/1 -> Bus Creator/32
  BSPR_uBattVolt/1 -> Bus Creator/30
  BCMR_flgTxBMT/1 -> Bus Creator/12
  BSPR_idxCellVoltMax/1 -> Bus Creator/21
  BCMR_stOtherErrBem/1 -> Bus Creator/49
  BCMR_bDChrgStopEna/1 -> Bus Creator/50
  BCMR_stDcBattSocErr/1 -> Bus Creator/51
  BCMR_stDChrgerActStop/1 -> Bus Creator/52
  BSER_pConstPwrDisCh/1 -> Bus Creator/53
  BCMR_verDChrgCom2015/1 -> Bus Creator/54
  BCMR_flgDChrgStopBActive/1 -> Bus Creator/55
  BCMR_flgDChrgStopCActive/1 -> Bus Creator/56
  BCMR_bDChrgWkup/1 -> Bus Creator/57

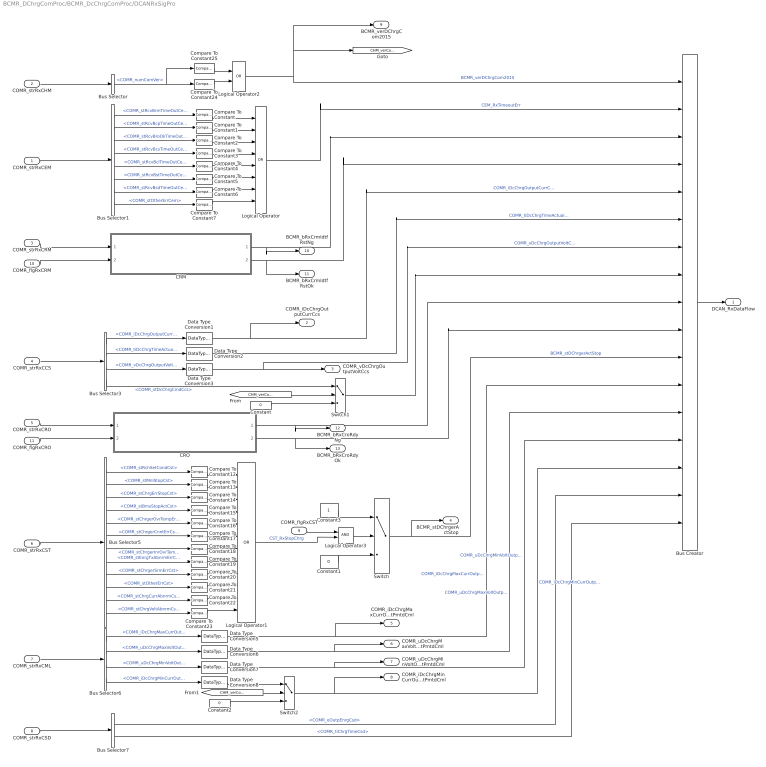
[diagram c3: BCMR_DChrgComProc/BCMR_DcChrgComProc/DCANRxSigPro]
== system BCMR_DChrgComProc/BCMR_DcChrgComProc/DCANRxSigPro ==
  COMR_strRxCEM : Inport  OutDataTypeStr=Bus: MSG_CEM_ERR
  COMR_strRxCHM : Inport  Port=2  OutDataTypeStr=Bus: MSG_CHM_P1
  COMR_strRxCRM : Inport  Port=3  OutDataTypeStr=Bus: MSG_CRM_P1
  COMR_strRxCCS : Inport  Port=4  OutDataTypeStr=Bus: MSG_CCS_P3
  COMR_strRxCRO : Inport  Port=5  OutDataTypeStr=Bus: MSG_CRO_P2
  COMR_strRxCST : Inport  Port=6  OutDataTypeStr=Bus: MSG_CST_P3
  COMR_strRxCML : Inport  Port=7  OutDataTypeStr=Bus: MSG_CML_P2
  COMR_strRxCSD : Inport  Port=8  OutDataTypeStr=Bus: MSG_CSD_P4
  COMR_flgRxCST : Inport  Port=9
  COMR_flgRxCRM : Inport  Port=10
  COMR_flgRxCRO : Inport  Port=11
  Bus Creator : BusCreator  Inputs=17
  Bus Selector : BusSelector  OutputSignals=COMR_numComVer
  Bus Selector1 : BusSelector  OutputSignals=COMR_stRcvBrmTimeOutCem,COMR_stRcvBcpTimeOutCem,COMR_stRcvBroOkTimeOutCem,COMR_stRcvBcsTimeOutCem,COMR_stRcvBclTimeOutCem,COMR_stRcvBstTimeOutCem,COMR_stRcvBsdTimeOutCem,COMR_stOtherErrCem
  Bus Selector3 : BusSelector  OutputSignals=COMR_iDcChrgOutputCurrCcs,COMR_tiDcChrgTimeActualCcs,COMR_vDcChrgOutputVoltCcs,COMR_stDcChrgCmdCcs
  Bus Selector5 : BusSelector  OutputSignals=COMR_stRchSetCondCst,COMR_stMnlStopCst,COMR_stChrgErrStopCst,COMR_stBmsStopActCst,COMR_stChrgerOvrTempErrCst,COMR_stChrgerCnntErrCst,COMR_stChrgerInrOvrTempErrCst,COMR_stEnrgTxAbnrmErrCst,COMR_stChrgerSrmErrCst,COMR_stOtherErrCst,COMR_stChrgCurrAbnrmCst,COMR_stChrgVoltAbnrmCst
  Bus Selector6 : BusSelector  OutputSignals=COMR_iDcChrgMaxCurrOutputPmtdCml,COMR_uDcChrgMaxVoltOutputPmtdCml,COMR_uDcChrgMinVoltOutputPmtdCml,COMR_iDcChrgMinCurrOutputPmtdCml
  Bus Selector7 : BusSelector  OutputSignals=COMR_eOutpEnrgCsd,COMR_tiChrgTimeCsd
  CRM : Subsystem
  CRO : Subsystem
  Compare To Constant{,1..7,12..23} (20 alike) : simulink/Logic and Bit Operations/Compare To Constant  relop===  const=1  OutDataTypeStr=boolean
  Compare To Constant24 : simulink/Logic and Bit Operations/Compare To Constant  relop===  const=257  OutDataTypeStr=boolean
  Compare To Constant25 : simulink/Logic and Bit Operations/Compare To Constant  relop===  const=2015  OutDataTypeStr=boolean
  Constant : Constant  Value=0  OutDataTypeStr=uint8
  Constant1 : Constant  Value=0  OutDataTypeStr=uint8
  Constant2 : Constant  Value=0  OutDataTypeStr=single
  Constant3 : Constant  OutDataTypeStr=uint8
  Data Type Conversion{1..3,5..8} (7 alike) : DataTypeConversion  OutDataTypeStr=single
  Logical Operator : Logic  Operator=OR  Inputs=8  AllPortsSameDT=off  OutDataTypeStr=boolean
  Logical Operator1 : Logic  Operator=OR  Inputs=12  AllPortsSameDT=off  OutDataTypeStr=boolean
  Logical Operator2 : Logic  Operator=OR  AllPortsSameDT=off  OutDataTypeStr=boolean
  Logical Operator3 : Logic  AllPortsSameDT=off  OutDataTypeStr=boolean
  Switch : Switch  Criteria=u2 > Threshold
  Switch1 : Switch  Criteria=u2 > Threshold
  Switch2 : Switch  Criteria=u2 > Threshold
  DCAN_RxDataFlow : Outport
  COMR_iDcChrgOutputCurrCcs : Outport  Port=2
  COMR_vDcChrgOutputVoltCcs : Outport  Port=3
  BCMR_stDChrgerActStop : Outport  Port=4
  COMR_iDcChrgMaxCurrOutputPmtdCml : Outport  Port=5
  COMR_uDcChrgMaxVoltOutputPmtdCml : Outport  Port=6
  COMR_uDcChrgMinVoltOutputPmtdCml : Outport  Port=7
  COMR_iDcChrgMinCurrOutputPmtdCml : Outport  Port=8
  BCMR_verDChrgCom2015 : Outport  Port=9
  BCMR_bRxCrmIdtfRstNg : Outport  Port=10
  BCMR_bRxCrmIdtfRstOk : Outport  Port=11
  BCMR_bRxCroRdyNg : Outport  Port=12
  BCMR_bRxCroRdyOk : Outport  Port=13
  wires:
  COMR_strRxCEM/1 -> Bus Selector1/1
  COMR_strRxCHM/1 -> Bus Selector/1
  Bus Selector1/1 -> Compare To Constant/1  "<COMR_stRcvBrmTimeOutCem>"
  Bus Selector1/2 -> Compare To Constant1/1  "<COMR_stRcvBcpTimeOutCem>"
  Bus Selector1/3 -> Compare To Constant2/1  "<COMR_stRcvBroOkTimeOutCem>"
  Bus Selector1/4 -> Compare To Constant3/1  "<COMR_stRcvBcsTimeOutCem>"
  Bus Selector1/5 -> Compare To Constant4/1  "<COMR_stRcvBclTimeOutCem>"
  Bus Selector1/6 -> Compare To Constant5/1  "<COMR_stRcvBstTimeOutCem>"
  Bus Selector1/7 -> Compare To Constant6/1  "<COMR_stRcvBsdTimeOutCem>"
  Bus Selector1/8 -> Compare To Constant7/1  "<COMR_stOtherErrCem>"
  Compare To Constant/1 -> Logical Operator/1
  Compare To Constant1/1 -> Logical Operator/2
  Compare To Constant2/1 -> Logical Operator/3
  Compare To Constant3/1 -> Logical Operator/4
  Compare To Constant4/1 -> Logical Operator/5
  Compare To Constant5/1 -> Logical Operator/6
  Compare To Constant6/1 -> Logical Operator/7
  Compare To Constant7/1 -> Logical Operator/8
  Logical Operator/1 -> Bus Creator/2  "CEM_RxTimeoutErr"
  COMR_strRxCST/1 -> Bus Selector5/1
  Bus Selector5/1 -> Compare To Constant12/1  "<COMR_stRchSetCondCst>"
  Bus Selector5/2 -> Compare To Constant13/1  "<COMR_stMnlStopCst>"
  Bus Selector5/3 -> Compare To Constant14/1  "<COMR_stChrgErrStopCst>"
  Bus Selector5/4 -> Compare To Constant15/1  "<COMR_stBmsStopActCst>"
  Bus Selector5/5 -> Compare To Constant16/1  "<COMR_stChrgerOvrTempErrCst>"
  Bus Selector5/6 -> Compare To Constant17/1  "<COMR_stChrgerCnntErrCst>"
  Bus Selector5/7 -> Compare To Constant18/1  "<COMR_stChrgerInrOvrTempErrCst>"
  Bus Selector5/8 -> Compare To Constant19/1  "<COMR_stEnrgTxAbnrmErrCst>"
  Bus Selector5/9 -> Compare To Constant20/1  "<COMR_stChrgerSrmErrCst>"
  Bus Selector5/10 -> Compare To Constant21/1  "<COMR_stOtherErrCst>"
  Bus Selector5/11 -> Compare To Constant22/1  "<COMR_stChrgCurrAbnrmCst>"
  Bus Selector5/12 -> Compare To Constant23/1  "<COMR_stChrgVoltAbnrmCst>"
  Compare To Constant12/1 -> Logical Operator1/1
  Compare To Constant13/1 -> Logical Operator1/2
  Compare To Constant14/1 -> Logical Operator1/3
  Compare To Constant15/1 -> Logical Operator1/4
  Compare To Constant16/1 -> Logical Operator1/5
  Compare To Constant17/1 -> Logical Operator1/6
  Compare To Constant18/1 -> Logical Operator1/7
  Compare To Constant19/1 -> Logical Operator1/8
  Compare To Constant20/1 -> Logical Operator1/9
  Compare To Constant21/1 -> Logical Operator1/10
  Compare To Constant22/1 -> Logical Operator1/11
  Compare To Constant23/1 -> Logical Operator1/12
  COMR_strRxCML/1 -> Bus Selector6/1
  COMR_strRxCSD/1 -> Bus Selector7/1
  Bus Selector7/1 -> Bus Creator/16  "<COMR_eOutpEnrgCsd>"
  Bus Selector7/2 -> Bus Creator/17  "<COMR_tiChrgTimeCsd>"
  Bus Selector/1 -> Compare To Constant25/1, Compare To Constant24/1  "<COMR_numComVer>"
  Constant3/1 -> Switch/1
  Constant1/1 -> Switch/3
  Switch/1 -> BCMR_stDChrgerActStop/1, Bus Creator/11  "BCMR_stDChrgerActStop"
  Bus Selector3/4 -> Switch1/1  "<COMR_stDcChrgCmdCcs>"
  Bus Selector3/3 -> Data Type Conversion3/1  "<COMR_vDcChrgOutputVoltCcs>"
  Bus Selector3/2 -> Data Type Conversion2/1  "<COMR_tiDcChrgTimeActualCcs>"
  Bus Selector3/1 -> Data Type Conversion1/1  "<COMR_iDcChrgOutputCurrCcs>"
  COMR_strRxCCS/1 -> Bus Selector3/1
  [CHM_verCom2015] -> Switch1/2
  Constant/1 -> Switch1/3
  [CHM_verCom2015] -> Switch2/2
  Constant2/1 -> Switch2/3
  Bus Selector6/4 -> Data Type Conversion8/1  "<COMR_iDcChrgMinCurrOutputPmtdCml>"
  Switch1/1 -> Bus Creator/8
  Bus Selector6/1 -> Data Type Conversion5/1  "<COMR_iDcChrgMaxCurrOutputPmtdCml>"
  Bus Selector6/2 -> Data Type Conversion6/1  "<COMR_uDcChrgMaxVoltOutputPmtdCml>"
  Bus Selector6/3 -> Data Type Conversion7/1  "<COMR_uDcChrgMinVoltOutputPmtdCml>"
  Switch2/1 -> COMR_iDcChrgMinCurrOutputPmtdCml/1, Bus Creator/15  "COMR_iDcChrgMinCurrOutputPmtdCml"
  Bus Creator/1 -> DCAN_RxDataFlow/1
  Compare To Constant25/1 -> Logical Operator2/1
  Compare To Constant24/1 -> Logical Operator2/2
  Logical Operator2/1 -> Bus Creator/1, BCMR_verDChrgCom2015/1, [CHM_verCom2015]  "BCMR_verDChrgCom2015"
  Data Type Conversion1/1 -> COMR_iDcChrgOutputCurrCcs/1, Bus Creator/5  "COMR_iDcChrgOutputCurrCcs"
  Data Type Conversion2/1 -> Bus Creator/6  "COMR_tiDcChrgTimeActualCcs"
  Data Type Conversion3/1 -> COMR_vDcChrgOutputVoltCcs/1, Bus Creator/7  "COMR_vDcChrgOutputVoltCcs"
  Data Type Conversion5/1 -> COMR_iDcChrgMaxCurrOutputPmtdCml/1, Bus Creator/12  "COMR_iDcChrgMaxCurrOutputPmtdCml"
  Data Type Conversion6/1 -> COMR_uDcChrgMaxVoltOutputPmtdCml/1, Bus Creator/13  "COMR_uDcChrgMaxVoltOutputPmtdCml"
  Data Type Conversion7/1 -> COMR_uDcChrgMinVoltOutputPmtdCml/1, Bus Creator/14  "COMR_uDcChrgMinVoltOutputPmtdCml"
  Data Type Conversion8/1 -> Switch2/1
  Logical Operator1/1 -> Logical Operator3/2  "CST_RxStopChrg"
  Logical Operator3/1 -> Switch/2
  COMR_flgRxCST/1 -> Logical Operator3/1
  COMR_strRxCRM/1 -> CRM/1(COMR_strRxCRM)
  COMR_flgRxCRM/1 -> CRM/2(COMR_flgRxCRM)
  CRM/1(BCMR_bRxCrmIdtfRstNg) -> BCMR_bRxCrmIdtfRstNg/1, Bus Creator/3
  CRM/2(BCMR_bRxCrmIdtfRstOk) -> BCMR_bRxCrmIdtfRstOk/1, Bus Creator/4
  COMR_strRxCRO/1 -> CRO/1(COMR_strRxCRO)
  COMR_flgRxCRO/1 -> CRO/2(COMR_flgRxCRO)
  CRO/1(BCMR_bRxCroRdyNg) -> Bus Creator/9, BCMR_bRxCroRdyNg/1
  CRO/2(BCMR_bRxCroRdyOk) -> Bus Creator/10, BCMR_bRxCroRdyOk/1

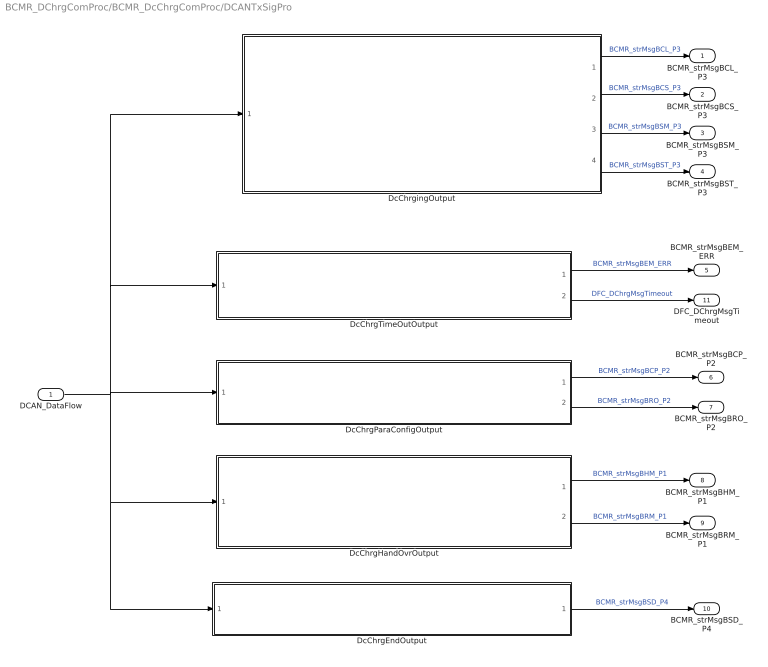
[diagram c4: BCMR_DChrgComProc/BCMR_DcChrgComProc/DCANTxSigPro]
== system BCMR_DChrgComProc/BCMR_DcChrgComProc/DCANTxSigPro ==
  DCAN_DataFlow : Inport
  DcChrgEndOutput : Subsystem
  DcChrgHandOvrOutput : Subsystem
  DcChrgParaConfigOutput : Subsystem
  DcChrgTimeOutOutput : Subsystem
  DcChrgingOutput : Subsystem
  BCMR_strMsgBCL_P3 : Outport  OutDataTypeStr=Bus: MSG_BCL_P3
  BCMR_strMsgBCS_P3 : Outport  Port=2  OutDataTypeStr=Bus: MSG_BCS_P3
  BCMR_strMsgBSM_P3 : Outport  Port=3  OutDataTypeStr=Bus: MSG_BSM_P3
  BCMR_strMsgBST_P3 : Outport  Port=4  OutDataTypeStr=Bus: MSG_BST_P3
  BCMR_strMsgBEM_ERR : Outport  Port=5  OutDataTypeStr=Bus: MSG_BEM_ERR
  BCMR_strMsgBCP_P2 : Outport  Port=6  OutDataTypeStr=Bus: MSG_BCP_P2
  BCMR_strMsgBRO_P2 : Outport  Port=7  OutDataTypeStr=Bus: MSG_BRO_P2
  BCMR_strMsgBHM_P1 : Outport  Port=8  OutDataTypeStr=Bus: MSG_BHM_P1
  BCMR_strMsgBRM_P1 : Outport  Port=9  OutDataTypeStr=Bus: MSG_BRM_P1
  BCMR_strMsgBSD_P4 : Outport  Port=10  OutDataTypeStr=Bus: MSG_BSD_P4
  DFC_DChrgMsgTimeout : Outport  Port=11
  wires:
  DcChrgingOutput/1("BCMR_strMsgBCL_P3 ") -> BCMR_strMsgBCL_P3/1  "BCMR_strMsgBCL_P3"
  DcChrgingOutput/2(BCMR_strMsgBCS_P3) -> BCMR_strMsgBCS_P3/1  "BCMR_strMsgBCS_P3"
  DcChrgingOutput/3(BCMR_strMsgBSM_P3) -> BCMR_strMsgBSM_P3/1  "BCMR_strMsgBSM_P3"
  DcChrgingOutput/4(BCMR_strMsgBST_P3) -> BCMR_strMsgBST_P3/1  "BCMR_strMsgBST_P3"
  DcChrgTimeOutOutput/1("BCMR_strMsgBEM_ERR ") -> BCMR_strMsgBEM_ERR/1  "BCMR_strMsgBEM_ERR"
  DcChrgParaConfigOutput/1("BCMR_strMsgBCP_P2 ") -> BCMR_strMsgBCP_P2/1  "BCMR_strMsgBCP_P2"
  DcChrgParaConfigOutput/2(BCMR_strMsgBRO_P2) -> BCMR_strMsgBRO_P2/1  "BCMR_strMsgBRO_P2"
  DcChrgHandOvrOutput/1("BCMR_strMsgBHM_P1 ") -> BCMR_strMsgBHM_P1/1  "BCMR_strMsgBHM_P1"
  DcChrgHandOvrOutput/2("BCMR_strMsgBRM_P1 ") -> BCMR_strMsgBRM_P1/1  "BCMR_strMsgBRM_P1"
  DcChrgEndOutput/1("BCMR_strMsgBSD_P4 ") -> BCMR_strMsgBSD_P4/1  "BCMR_strMsgBSD_P4"
  DCAN_DataFlow/1 -> DcChrgEndOutput/1(DCAN_DataFlow), DcChrgHandOvrOutput/1(DCAN_DataFlow), DcChrgingOutput/1(DCAN_DataFlow), DcChrgTimeOutOutput/1(DCAN_DataFlow), DcChrgParaConfigOutput/1(DCAN_DataFlow)
  DcChrgTimeOutOutput/2(DFC_DChrgMsgTimeout) -> DFC_DChrgMsgTimeout/1  "DFC_DChrgMsgTimeout"

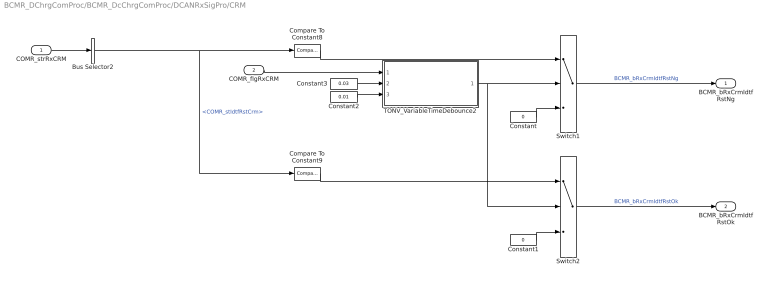
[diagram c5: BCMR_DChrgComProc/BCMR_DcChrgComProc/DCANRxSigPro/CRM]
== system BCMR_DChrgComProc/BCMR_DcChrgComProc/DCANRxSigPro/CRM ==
  COMR_strRxCRM : Inport  OutDataTypeStr=Bus: MSG_CRM_P1
  COMR_flgRxCRM : Inport  Port=2
  Bus Selector2 : BusSelector  OutputSignals=COMR_stIdtfRstCrm
  Compare To Constant8 : simulink/Logic and Bit Operations/Compare To Constant  relop===  const=0  OutDataTypeStr=boolean
  Compare To Constant9 : simulink/Logic and Bit Operations/Compare To Constant  relop===  const=170  OutDataTypeStr=boolean
  Constant : Constant  Value=0  OutDataTypeStr=boolean
  Constant1 : Constant  Value=0  OutDataTypeStr=boolean
  Constant2 : Constant  Value=0.01  OutDataTypeStr=single
  Constant3 : Constant  Value=0.03  OutDataTypeStr=single
  Switch1 : Switch  Criteria=u2 ~= 0
  Switch2 : Switch  Criteria=u2 ~= 0
  TONV_VariableTimeDebounce2 : Subsystem  TreatAsAtomicUnit=on  RTWFcnName=TONV_VariableTimeDebounce  RTWFileName=SrvLib
  BCMR_bRxCrmIdtfRstNg : Outport
  BCMR_bRxCrmIdtfRstOk : Outport  Port=2
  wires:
  Bus Selector2/1 -> Compare To Constant9/1, Compare To Constant8/1  "<COMR_stIdtfRstCrm>"
  COMR_strRxCRM/1 -> Bus Selector2/1
  Compare To Constant8/1 -> Switch1/1
  COMR_flgRxCRM/1 -> TONV_VariableTimeDebounce2/1(u)
  Constant/1 -> Switch1/3
  Switch1/1 -> BCMR_bRxCrmIdtfRstNg/1  "BCMR_bRxCrmIdtfRstNg"
  Compare To Constant9/1 -> Switch2/1
  Constant1/1 -> Switch2/3
  Switch2/1 -> BCMR_bRxCrmIdtfRstOk/1  "BCMR_bRxCrmIdtfRstOk"
  TONV_VariableTimeDebounce2/1(y) -> Switch2/2, Switch1/2
  Constant2/1 -> TONV_VariableTimeDebounce2/3(dT)
  Constant3/1 -> TONV_VariableTimeDebounce2/2(T)

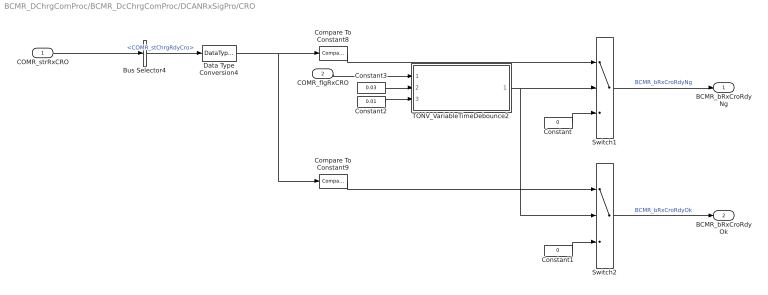
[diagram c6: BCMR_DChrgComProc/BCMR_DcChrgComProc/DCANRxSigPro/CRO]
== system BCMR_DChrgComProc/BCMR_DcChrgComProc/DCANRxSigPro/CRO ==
  COMR_strRxCRO : Inport  OutDataTypeStr=Bus: MSG_CRO_P2
  COMR_flgRxCRO : Inport  Port=2
  Bus Selector4 : BusSelector  OutputSignals=COMR_stChrgRdyCro
  Compare To Constant8 : simulink/Logic and Bit Operations/Compare To Constant  relop===  const=0  OutDataTypeStr=boolean
  Compare To Constant9 : simulink/Logic and Bit Operations/Compare To Constant  relop===  const=170  OutDataTypeStr=boolean
  Constant : Constant  Value=0  OutDataTypeStr=boolean
  Constant1 : Constant  Value=0  OutDataTypeStr=boolean
  Constant2 : Constant  Value=0.01  OutDataTypeStr=single
  Constant3 : Constant  Value=0.03  OutDataTypeStr=single
  Data Type Conversion4 : DataTypeConversion
  Switch1 : Switch  Criteria=u2 ~= 0
  Switch2 : Switch  Criteria=u2 ~= 0
  TONV_VariableTimeDebounce2 : Subsystem  TreatAsAtomicUnit=on  RTWFcnName=TONV_VariableTimeDebounce  RTWFileName=SrvLib
  BCMR_bRxCroRdyNg : Outport
  BCMR_bRxCroRdyOk : Outport  Port=2
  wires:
  COMR_strRxCRO/1 -> Bus Selector4/1
  Bus Selector4/1 -> Data Type Conversion4/1  "<COMR_stChrgRdyCro>"
  Compare To Constant8/1 -> Switch1/1
  COMR_flgRxCRO/1 -> TONV_VariableTimeDebounce2/1(u)
  Constant/1 -> Switch1/3
  Compare To Constant9/1 -> Switch2/1
  Constant1/1 -> Switch2/3
  TONV_VariableTimeDebounce2/1(y) -> Switch2/2, Switch1/2
  Constant2/1 -> TONV_VariableTimeDebounce2/3(dT)
  Constant3/1 -> TONV_VariableTimeDebounce2/2(T)
  Data Type Conversion4/1 -> Compare To Constant9/1, Compare To Constant8/1
  Switch1/1 -> BCMR_bRxCroRdyNg/1  "BCMR_bRxCroRdyNg"
  Switch2/1 -> BCMR_bRxCroRdyOk/1  "BCMR_bRxCroRdyOk"

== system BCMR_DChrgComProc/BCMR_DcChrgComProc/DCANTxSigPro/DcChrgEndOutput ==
  DCAN_DataFlow : Inport
  Bus Selector : BusSelector  OutputSignals=BCMR_flgTxBSD,BSPR_tCellTempMax,BSPR_tCellTempMin,BSPR_uCellVoltMin,BSPR_uCellVoltMax,BSER_rSocDspl
  Data Type Conversion : DataTypeConversion  OutDataTypeStr=uint8
  Terminator1 : Terminator
  TxBSD : Subsystem
  "BCMR_strMsgBSD_P4 " : Outport  OutDataTypeStr=Bus: MSG_BSD_P4
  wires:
  TxBSD/1("BCMR_strMsgBSD_P4 ") -> "BCMR_strMsgBSD_P4 "/1  "BCMR_strMsgBSD_P4"
  DCAN_DataFlow/1 -> Bus Selector/1
  Bus Selector/2 -> TxBSD/1(BCMR_tBattMaxTempBsd)  "<BSPR_tCellTempMax>"
  Bus Selector/3 -> TxBSD/2(BCMR_tBattMinTempBsd)  "<BSPR_tCellTempMin>"
  Bus Selector/4 -> TxBSD/3(BCMR_vBattMinCellVoltBsd)  "<BSPR_uCellVoltMin>"
  Bus Selector/5 -> TxBSD/4(BCMR_vBattMaxCellVoltBsd)  "<BSPR_uCellVoltMax>"
  Bus Selector/6 -> Data Type Conversion/1  "<BSER_rSocDspl>"
  Data Type Conversion/1 -> TxBSD/5(BCMR_rBattSocBsd)
  Bus Selector/1 -> Terminator1/1  "<BCMR_flgTxBSD>"

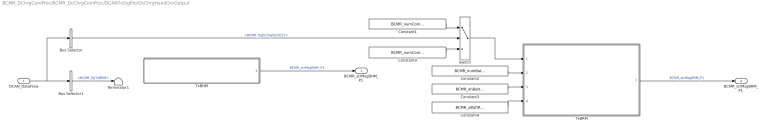
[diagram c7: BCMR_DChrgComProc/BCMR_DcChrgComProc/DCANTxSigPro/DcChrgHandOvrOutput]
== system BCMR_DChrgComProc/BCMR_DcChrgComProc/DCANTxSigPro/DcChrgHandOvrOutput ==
  DCAN_DataFlow : Inport
  Bus Selector : BusSelector  OutputSignals=BCMR_flgDChrgVer2015
  Bus Selector1 : BusSelector  OutputSignals=BCMR_flgTxBRM
  Constant1 : Constant  Value=BCMR_numComVer2015Brm_C
  Constant2 : Constant  Value=BCMR_numBattTypeBrm_C
  Constant3 : Constant  Value=BCMR_ahBattRatdCpctyBrm_C
  Constant4 : Constant  Value=BCMR_uBattRatdPackVoltBrm_C
  Constant9 : Constant  Value=BCMR_numComVer2011Brm_C
  Switch : Switch  Criteria=u2 > Threshold
  Terminator1 : Terminator
  TxBHM : Subsystem
  TxBRM : Subsystem
  "BCMR_strMsgBHM_P1 " : Outport  OutDataTypeStr=Bus: MSG_BHM_P1
  "BCMR_strMsgBRM_P1 " : Outport  Port=2  OutDataTypeStr=Bus: MSG_BRM_P1
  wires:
  TxBHM/1("BCMR_strMsgBHM_P1 ") -> "BCMR_strMsgBHM_P1 "/1  "BCMR_strMsgBHM_P1"
  TxBRM/1("BCMR_strMsgBRM_P1 ") -> "BCMR_strMsgBRM_P1 "/1  "BCMR_strMsgBRM_P1"
  DCAN_DataFlow/1 -> Bus Selector1/1, Bus Selector/1
  Constant2/1 -> TxBRM/2(BCMR_numBattTypeBrm)
  Constant3/1 -> TxBRM/3(BCMR_ahBattRatdCpctyBrm)
  Constant4/1 -> TxBRM/4(BCMR_uBattRatdPackVoltBrm)
  Bus Selector/1 -> Switch/2  "<BCMR_flgDChrgVer2015>"
  Bus Selector1/1 -> Terminator1/1  "<BCMR_flgTxBRM>"
  Constant9/1 -> Switch/3
  Constant1/1 -> Switch/1
  Switch/1 -> TxBRM/1(BCMR_numComVerBrm)

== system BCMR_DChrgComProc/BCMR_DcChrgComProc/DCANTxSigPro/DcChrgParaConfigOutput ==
  DCAN_DataFlow : Inport
  Bus Selector : BusSelector  OutputSignals=BCMR_flgTxBCP,BSER_rSocDspl,BSPR_uBattVolt,BCMR_bDChrgWkup
  Bus Selector1 : BusSelector  OutputSignals=BCMR_flgTxBRO,BCMR_stBmsRdyBro
  Constant5 : Constant  Value=BCMR_uMaxChrgCellVoltPmtdBcp_C
  Constant6 : Constant  Value=BCMR_eBattRatedEnrgBcp_C
  Constant7 : Constant  Value=BCMR_uBattRatdPackVoltBcp_C
  Constant8 : Constant  Value=BCMR_tMaxTempPmtdBcp_C
  Constant9 : Constant  Value=BCMR_iMaxChrgCurrPmtdBcp_C
  Terminator1 : Terminator
  Terminator2 : Terminator
  TxBCP : Subsystem
  TxBRO : Subsystem
  "BCMR_strMsgBCP_P2 " : Outport  OutDataTypeStr=Bus: MSG_BCP_P2
  BCMR_strMsgBRO_P2 : Outport  Port=2  OutDataTypeStr=Bus: MSG_BRO_P2
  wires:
  TxBCP/1("BCMR_strMsgBCP_P2 ") -> "BCMR_strMsgBCP_P2 "/1  "BCMR_strMsgBCP_P2"
  TxBRO/1(BCMR_strMsgBRO_P2) -> BCMR_strMsgBRO_P2/1  "BCMR_strMsgBRO_P2"
  DCAN_DataFlow/1 -> Bus Selector1/1, Bus Selector/1
  Bus Selector1/2 -> TxBRO/1(BCMR_stBmsRdyBro)  "<BCMR_stBmsRdyBro>"
  Constant5/1 -> TxBCP/4(BCMR_vMaxChrgCellVoltPmtdBcp)
  Constant9/1 -> TxBCP/5(BCMR_iMaxChrgCurrPmtdBcp)
  Constant6/1 -> TxBCP/6(BCMR_eBattRatedEnrgBcp)
  Constant7/1 -> TxBCP/7(BCMR_uBattRatdPackVoltBcp)
  Constant8/1 -> TxBCP/8(BCMR_cMaxTempPmtdBcp)
  Bus Selector/2 -> TxBCP/1(BCMR_rSocDsplBcp)  "<BSER_rSocDspl>"
  Bus Selector/3 -> TxBCP/2(BCMR_uBattVoltBcp)  "<BSPR_uBattVolt>"
  Bus Selector/1 -> Terminator1/1  "<BCMR_flgTxBCP>"
  Bus Selector1/1 -> Terminator2/1  "<BCMR_flgTxBRO>"
  Bus Selector/4 -> TxBCP/3(BCMR_bDChrgWkup)  "<BCMR_bDChrgWkup>"

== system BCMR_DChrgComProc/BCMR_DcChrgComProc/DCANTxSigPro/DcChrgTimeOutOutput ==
  DCAN_DataFlow : Inport
  Bus Selector : BusSelector  OutputSignals=BCMR_flgTxBEM,BCMR_stSpn3901TimeoutBem,BCMR_stSpn3902TimeoutBem,BCMR_stSpn3903TimeoutBem,BCMR_stSpn3904TimeoutBem,BCMR_stSpn3905TimeoutBem,BCMR_stSpn3906TimeoutBem,BCMR_stSpn3907TimeoutBem,BCMR_stOtherErrBem
  DSM_ReportCheck : Subsystem  TreatAsAtomicUnit=on  RTWFcnName=DSM_ReportCheck  RTWFileName=SrvLib
  Delay : Delay  DelayLength=1  InitialCondition=0
  Logical Operator2 : Logic  Operator=NOT  AllPortsSameDT=off  OutDataTypeStr=boolean
  TxBEM : Subsystem
  "BCMR_strMsgBEM_ERR " : Outport  OutDataTypeStr=Bus: MSG_BEM_ERR
  DFC_DChrgMsgTimeout : Outport  Port=2
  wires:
  TxBEM/1("BCMR_strMsgBEM_ERR ") -> "BCMR_strMsgBEM_ERR "/1  "BCMR_strMsgBEM_ERR"
  DCAN_DataFlow/1 -> Bus Selector/1
  Bus Selector/2 -> TxBEM/1(BCMR_stSpn3901TimeoutBem)  "<BCMR_stSpn3901TimeoutBem>"
  Bus Selector/3 -> TxBEM/2(BCMR_stSpn3902TimeoutBem)  "<BCMR_stSpn3902TimeoutBem>"
  Bus Selector/4 -> TxBEM/3(BCMR_stSpn3903TimeoutBem)  "<BCMR_stSpn3903TimeoutBem>"
  Bus Selector/5 -> TxBEM/4(BCMR_stSpn3904TimeoutBem)  "<BCMR_stSpn3904TimeoutBem>"
  Bus Selector/6 -> TxBEM/5(BCMR_stSpn3905TimeoutBem)  "<BCMR_stSpn3905TimeoutBem>"
  Bus Selector/7 -> TxBEM/6(BCMR_stSpn3906TimeoutBem)  "<BCMR_stSpn3906TimeoutBem>"
  Bus Selector/8 -> TxBEM/7(BCMR_stSpn3907TimeoutBem)  "<BCMR_stSpn3907TimeoutBem>"
  Bus Selector/1 -> DSM_ReportCheck/2(Err), Logical Operator2/1  "<BCMR_flgTxBEM>"
  Bus Selector/9 -> TxBEM/8(BCMR_stOtherErrBem)  "<BCMR_stOtherErrBem>"
  Delay/1 -> DSM_ReportCheck/1(Dfc_id_nv)
  Logical Operator2/1 -> DSM_ReportCheck/3(Heal)
  DSM_ReportCheck/1(Dfc_id) -> DFC_DChrgMsgTimeout/1, Delay/1  "DFC_DChrgMsgTimeout"
